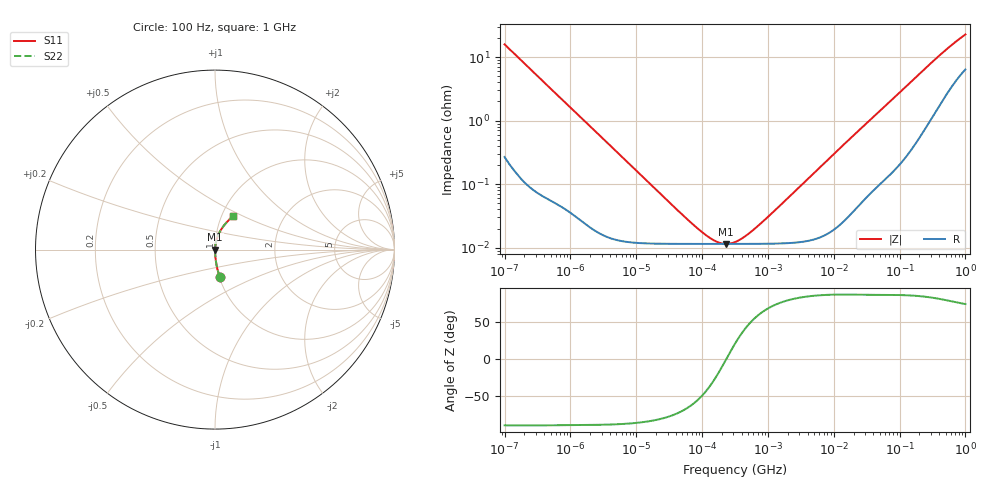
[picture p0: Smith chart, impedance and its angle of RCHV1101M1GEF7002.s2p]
! RCHV1101M1GEF7002  S-PARAMETER MODEL  (AEC-Q200 qualified)
! Model Generated by ELNA Corporation (http://www.ty-top.com)
! Version 1.0
! ELNA Control No. 240229
! Copyright (c) 2024 ELNA CO.,LTD. All Rights Reserved.
! Products Name : CONDUCTIVE POLYMER HYBRID ALUMINUM ELECTROLYTIC CAPACITORS
! Characteristics :
!  Capacitance  :  100uF  ,  Rated voltage  :  35V
!  Operating Temp. Range  :  -55 to +105 degC  ,  Endurance  :  5000hr at 105 degC
!  Dimension D  :  8mm  ,  Dimension L  :  8.7mm
! Frequency Range : 100Hz - 1GHz
! External Node Assignments :
!  1  o---| |---o  2
# MHz S RI R 50
!Freq[MHz].  S11 Real  S11 Imag  S21 Real  S21 Imag  S12 Real  S12 Imag  S22 Real  S22 Imag
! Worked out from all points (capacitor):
!   401 points, 100 Hz to 1 GHz, reference 50 ohm
!   read as one part in series: C = 100 uF near 108 Hz
!   lowest |Z| = 11.5 mohm at 229.1 kHz (marker M1)
!   series resonance near 233.6 kHz, so ESL is about 4.6 nH
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0.0001  0.027 -0.1537  0.973 0.1537  0.973 0.1537  0.027 -0.1537
0.000113  0.0214 -0.1371  0.9786 0.1371  0.9786 0.1371  0.0214 -0.1371
0.000183  0.00859 -0.0858  0.9914 0.0858  0.9914 0.0858  0.00859 -0.0858
0.000309  0.00336 -0.0512  0.9966 0.0512  0.9966 0.0512  0.00336 -0.0512
0.001488  0.000377 -0.0108  0.9996 0.0108  0.9996 0.0108  0.000377 -0.0108
0.022131  0.000116 -0.000729  0.9999 0.000729  0.9999 0.000729  0.000116 -0.000729
0.060604  0.000115 -0.00025  0.9999 0.00025  0.9999 0.00025  0.000115 -0.00025
0.106537  0.000115 -0.000121  0.9999 0.000121  0.9999 0.000121  0.000115 -0.000121
0.159404  0.000115 -5.45e-05  0.9999 5.45e-05  0.9999 5.45e-05  0.000115 -5.45e-05
0.194984  0.000115 -2.53e-05  0.9999 2.53e-05  0.9999 2.53e-05  0.000115 -2.53e-05
0.229087  0.000115 -2.67e-06  0.9999 2.67e-06  0.9999 2.67e-06  0.000115 -2.67e-06
0.269153  0.000115 1.99e-05  0.9999 -1.99e-05  0.9999 -1.99e-05  0.000115 1.99e-05
0.316228  0.000115 4.29e-05  0.9999 -4.29e-05  0.9999 -4.29e-05  0.000115 4.29e-05
0.454465  0.000115 9.98e-05  0.9999 -9.98e-05  0.9999 -9.98e-05  0.000115 9.98e-05
0.707946  0.000115 0.000188  0.9999 -0.000188  0.9999 -0.000188  0.000115 0.000188
4.704354  0.000134 0.0014  0.9999 -0.0014  0.9999 -0.0014  0.000134 0.0014
17.08048  0.000339 0.00501  0.9997 -0.00501  0.9997 -0.00501  0.000339 0.00501
69.9842  0.00175 0.0194  0.9983 -0.0194  0.9983 -0.0194  0.00175 0.0194
176.8072  0.00665 0.0474  0.9933 -0.0474  0.9933 -0.0474  0.00665 0.0474
395.8221  0.0263 0.0984  0.9737 -0.0984  0.9737 -0.0984  0.0263 0.0984
668.3439  0.0592 0.1456  0.9408 -0.1456  0.9408 -0.1456  0.0592 0.1456
1000  0.0977 0.1845  0.9023 -0.1845  0.9023 -0.1845  0.0977 0.1845
